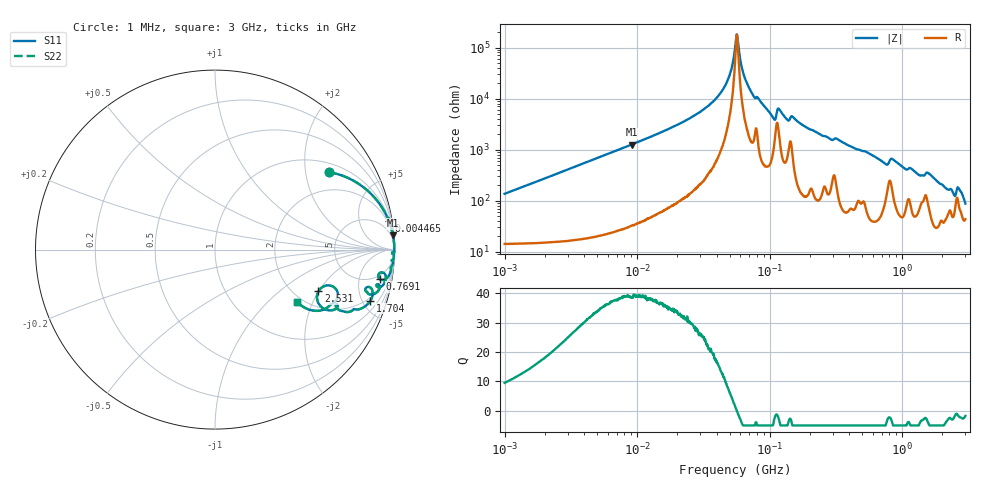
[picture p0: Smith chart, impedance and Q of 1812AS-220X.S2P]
!s-Parameter Generated by FASTRON Sdn. Bhd.
!FASTRON P/N : 1812AS-220X
!Keysight Technologies,E4991B,MY54100416,A.01.15
!Date created: Mon Oct 16 09:56:26 2023
!Version  : Rev00 Mon Oct 16 09:56:26 2023
!Data & Calibration Information:
!Freq	S11	S21	S12	S22
!PortZ  Port1:50+j0  Port2:50+j0
!When reading, reference impedance value at option line is always used.
! Remarks : This data is being provided solely for informational purposes.
# Hz S dB R 50
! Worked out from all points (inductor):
!   1601 points, 1 MHz to 3 GHz, reference 50 ohm
!   read as one part in series: L = 21.5 uH near 1.041 MHz
!   highest Q = 39.2 at 9.086 MHz (marker M1), where L = 22 uH
!   self-resonance near 56.44 MHz
!   S11 on the Smith chart (normalised r, x): 1 MHz: 1.28, +2.71; 4.465 MHz: 1, +12; 769.1 MHz: 4, -10; 1.704 GHz: 1.71, -5.76; 2.531 GHz: 2.63, -1.99; 3 GHz: 1.87, -1.53
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1000000  -2.28 34.1  -4.97 -49.9  -4.97 -49.9  -2.28 34.1
3804036  -0.21 10.9  -14.47 -77.2  -14.47 -77.2  -0.21 10.9
4464646  -0.16 9.3  -15.82 -78.9  -15.82 -78.9  -0.16 9.3
9086184  -0.05 4.5  -22.01 -84.0  -22.01 -84.0  -0.05 4.5
1.447069e7  -0.02 2.8  -26.35 -85.7  -26.35 -85.7  -0.02 2.8
3.936673e7  -0.01 0.6  -40.01 -86.0  -40.01 -86.0  -0.01 0.6
4.881767e7  -0.00 0.2  -47.85 -82.1  -47.85 -82.1  -0.00 0.2
5.477226e7  -0.00 0.1  -59.74 -58.0  -59.74 -58.0  -0.00 0.1
5.729536e7  -0.00 -0.0  -63.48 33.7  -63.48 33.7  -0.00 -0.0
6.33262e7  -0.01 -0.2  -49.85 79.2  -49.85 79.2  -0.01 -0.2
7.248696e7  -0.01 -0.4  -42.68 83.5  -42.68 83.5  -0.01 -0.4
1.060286e8  -0.04 -1.3  -32.59 77.1  -32.59 77.1  -0.04 -1.3
1.183678e8  -0.04 -0.9  -35.81 73.1  -35.81 73.1  -0.04 -0.9
1.354909e8  -0.04 -1.5  -31.80 78.5  -31.80 78.5  -0.04 -1.5
1.497525e8  -0.03 -1.3  -32.83 80.0  -32.83 80.0  -0.03 -1.3
2.083556e8  -0.03 -2.3  -27.75 83.7  -27.75 83.7  -0.03 -2.3
7.691493e8  -0.61 -10.1  -14.72 63.3  -14.72 63.3  -0.61 -10.1
7.925923e8  -0.71 -8.8  -15.55 57.5  -15.55 57.5  -0.71 -8.8
1.704314e9  -0.80 -18.2  -10.06 64.8  -10.06 64.8  -0.80 -18.2
2.530652e9  -4.14 -21.9  -6.32 28.7  -6.32 28.7  -4.14 -21.9
2.727913e9  -2.84 -24.5  -6.83 41.0  -6.83 41.0  -2.84 -24.5
3e9  -5.33 -32.4  -4.22 28.1  -4.22 28.1  -5.33 -32.4
